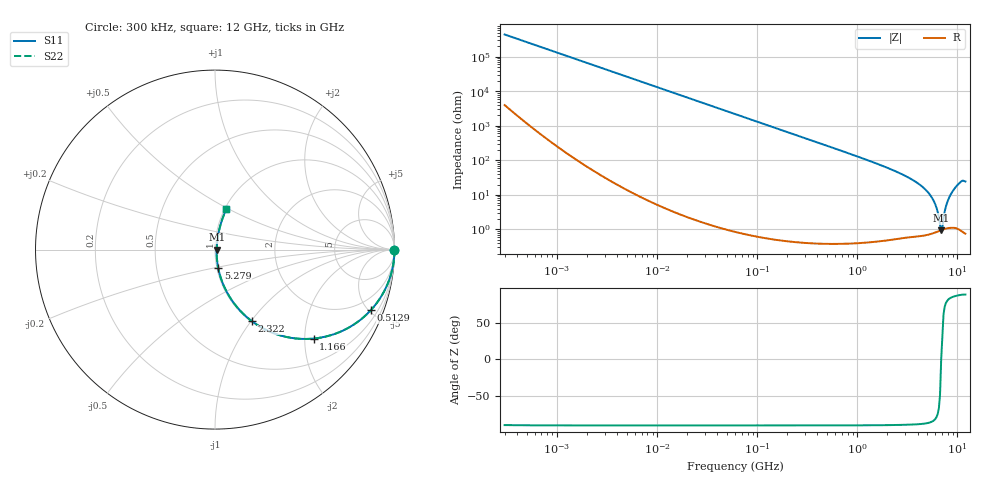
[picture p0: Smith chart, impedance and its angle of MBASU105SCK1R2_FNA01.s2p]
! MBASU105SCK1R2_FNA01  S-PARAMETER MODEL  ( Standard Model )
! Model Generated by TAIYO YUDEN Corporation (http://www.ty-top.com)
! Version 1.0
! TAIYO YUDEN Control No. 230609
! Copyright(c) 2023 TAIYO YUDEN CO.,LTD. All Rights Reserved.
! Product Description (link to TY-COMPAS)
! https://ds.yuden.co.jp/TYCOMPAS/or/detail?pn=MBASU105SCK1R2CFNA01&u=M
! Products Name : Multilayer Ceramic Capacitors
! Characteristics :
!  Capacitance : 1.2 [pF] , Rated Voltage : 50 [V] , TCC : CK / C0K
!  Case Size : 1.0 x 0.5 / 0.039 x 0.02 [mm/inch] , Thickness : 0.5 / 0.02 [mm/inch]
!  (Conditions: Temperature = 25 [degC] , DC Bias Voltage = 0 [V])
! External Node Assignments :
!  1  o---| |---o  2
! GND o---------o GND
! Frequency Range : 0.3MHz  -  12000MHz  [ 401 STEP ]
# MHZ S RI R 50
! Freq[MHz].  S11 Real  S11 Imag  S21 Real  S21 Imag  S12 Real  S12 Imag  S22 Real  S22 Imag
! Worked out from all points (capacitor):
!   401 points, 300 kHz to 12 GHz, reference 50 ohm
!   read as one part in series: C = 1.2 pF near 316.3 kHz
!   lowest |Z| = 948 mohm at 6.88 GHz (marker M1)
!   series resonance near 6.879 GHz, so ESL is about 450 pH
!   S11 on the Smith chart (normalised r, x): 300 kHz: open; 512.9 MHz: 1.01, -5.14; 1.166 GHz: 1.01, -2.21; 2.322 GHz: 1.01, -1.01; 5.279 GHz: 1.01, -0.21; 12 GHz: 1.02, +0.49
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0.3  1 -0.000226  2.09e-06 0.000226  2.09e-06 0.000226  1 -0.000226
1.769972  1 -0.00133  3.24e-06 0.00133  3.24e-06 0.00133  1 -0.00133
10.44266  0.9999 -0.00787  6.5e-05 0.00787  6.5e-05 0.00787  0.9999 -0.00787
60  0.9979 -0.0451  0.00206 0.0451  0.00206 0.0451  0.9979 -0.0451
159.8975  0.9856 -0.1189  0.0144 0.1189  0.0144 0.1189  0.9856 -0.1189
353.9943  0.9329 -0.2496  0.0671 0.2496  0.0671 0.2496  0.9329 -0.2496
512.9422  0.8683 -0.3375  0.1317 0.3375  0.1317 0.3375  0.8683 -0.3375
1166.079  0.5494 -0.4957  0.4506 0.4957  0.4506 0.4957  0.5494 -0.4957
2088.533  0.2513 -0.4295  0.7487 0.4295  0.7487 0.4295  0.2513 -0.4295
2321.999  0.2063 -0.3996  0.7937 0.3996  0.7937 0.3996  0.2063 -0.3996
3841.137  0.0586 -0.2223  0.9414 0.2223  0.9414 0.2223  0.0586 -0.2223
4623.766  0.0303 -0.1515  0.9697 0.1515  0.9697 0.1515  0.0303 -0.1515
5278.635  0.0175 -0.1007  0.9825 0.1007  0.9825 0.1007  0.0175 -0.1007
6026.253  0.0106 -0.0502  0.9894 0.0502  0.9894 0.0502  0.0106 -0.0502
6699.894  0.00922 -0.00994  0.9908 0.00994  0.9908 0.00994  0.00922 -0.00994
6879.757  0.0094 5.93e-05  0.9906 -5.93e-05  0.9906 -5.93e-05  0.0094 5.93e-05
7064.448  0.00971 0.00563  0.9903 -0.00563  0.9903 -0.00563  0.00971 0.00563
7254.098  0.0103 0.0178  0.9897 -0.0178  0.9897 -0.0178  0.0103 0.0178
7854.144  0.0138 0.0555  0.9862 -0.0555  0.9862 -0.0555  0.0138 0.0555
8732.115  0.0233 0.1095  0.9767 -0.1095  0.9767 -0.1095  0.0233 0.1095
10511.28  0.0557 0.2085  0.9443 -0.2085  0.9443 -0.2085  0.0557 0.2085
12000  0.0628 0.2276  0.9372 -0.2276  0.9372 -0.2276  0.0628 0.2276
